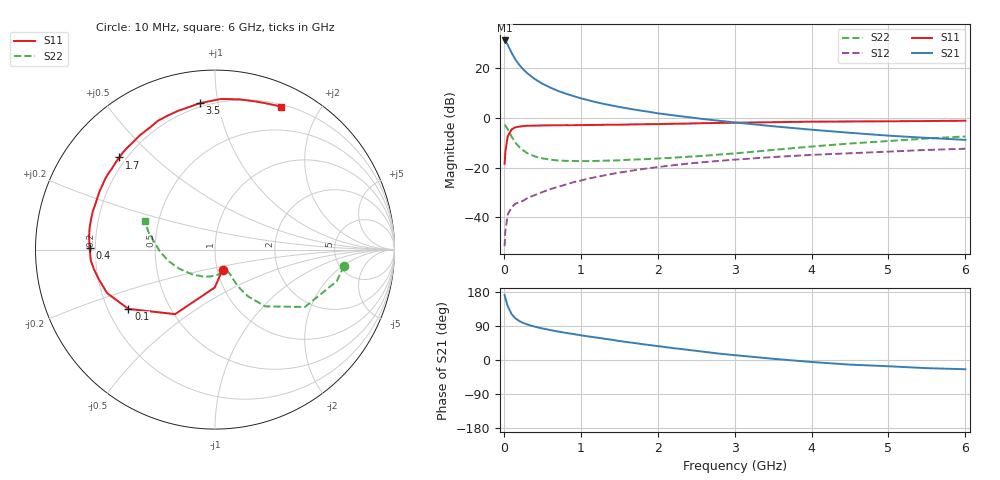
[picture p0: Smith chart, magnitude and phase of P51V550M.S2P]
! SIEMENS Small Signal Semiconductors
! BFP183
! Si NPN RF Bipolar Junction Transistor in SOT143
! VCE = 1.5 V  IC = 50 mA
! Common Emitter S-Parameters:  March  1996
# GHz  S  MA  R  50
!  f  S11  S21  S12  S22
! GHz  MAG  ANG  MAG  ANG  MAG  ANG  MAG  ANG
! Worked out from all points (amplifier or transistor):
!   36 points, 10 MHz to 6 GHz, reference 50 ohm
!   highest |S21| = 31.2 dB at 10 MHz (marker M1)
!   |S21| within 3 dB of that: start of sweep to 69.72 MHz
!   unconditionally stable (mu >= 1): start of sweep to 29.73 MHz; 188.7 MHz to end of sweep
!   at 250 MHz: K = 1.19, MAG = 23.9 dB, |S12| = -33.4 dB
!   at 1.4 GHz: K = 1.73, MAG = 8.8 dB, |S12| = -22.6 dB
!   at 6 GHz: K = 1.34, MAG = -1.7 dB, |S12| = -12.4 dB
!   S11 on the Smith chart (normalised r, x): 10 MHz: 1.06, -0.24; 100 MHz: 0.29, -0.29; 400 MHz: 0.18, +0.01; 1.7 GHz: 0.17, +0.39; 3.5 GHz: 0.18, +0.89; 6 GHz: 0.22, +1.54
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0.01  0.1192 -69.0  36.44 171.5  0.0026 68.7  0.7242 -7.1
0.02  0.2115 -90.5  35.46 163.3  0.0052 69.4  0.7012 -14.5
0.05  0.4226 -121.7  29.87 142.2  0.0113 60.1  0.5945 -32.5
0.1  0.5849 -145.6  20.59 121.4  0.0156 46.0  0.4224 -48.5
0.15  0.648 -158.0  15.1 110.0  0.0187 45.0  0.3184 -54.8
0.2  0.6678 -165.6  11.78 102.9  0.0201 45.0  0.2592 -57.3
0.25  0.6833 -170.8  9.59 97.9  0.0213 46.6  0.2228 -58.2
0.3  0.6946 -175.0  8.071 94.1  0.0239 49.2  0.1965 -58.5
0.4  0.699 179.1  6.125 88.0  0.0278 53.3  0.1681 -58.5
0.5  0.7055 174.1  4.903 83.3  0.032 55.1  0.153 -59.0
0.6  0.7093 170.0  4.123 79.2  0.0364 57.5  0.1445 -60.0
0.7  0.711 166.1  3.52 75.3  0.0407 58.9  0.1389 -61.6
0.9  0.7128 159.6  2.773 68.7  0.0504 60.1  0.1356 -65.7
1.1  0.7208 153.1  2.27 62.2  0.0599 60.1  0.1351 -70.9
1.3  0.7274 147.5  1.915 56.3  0.0691 59.2  0.1374 -76.9
1.7  0.7403 136.1  1.472 44.7  0.0883 56.5  0.1449 -89.8
2.2  0.762 123.4  1.132 31.4  0.1112 51.7  0.1576 -107.9
2.8  0.792 109.2  0.877 16.8  0.1362 45.0  0.1831 -129.3
3.5  0.8203 95.8  0.68 3.2  0.1626 37.7  0.2265 -152.1
4.5  0.8481 80.7  0.501 -12.2  0.1941 26.9  0.3052 -177.4
5.5  0.8652 69.8  0.396 -21.5  0.2266 17.5  0.3851 164.9
6  0.8783 65.1  0.361 -24.4  0.2392 12.2  0.4235 157.6
